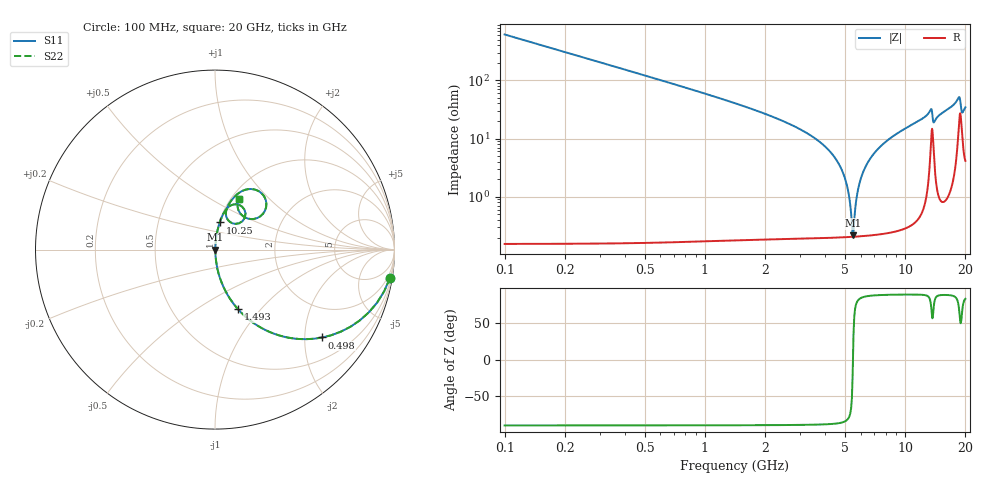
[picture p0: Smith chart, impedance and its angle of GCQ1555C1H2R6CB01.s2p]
!Murata Part Number: GCQ1555C1H2R6CB01
!These Parameters are Measured in Series Mode Connection
!Data Generated on Jan 08, 2026
!  o--ll--o
!Port1  Port2
!  o------o
!Operation Temp=25[degC], DC Bias Voltage=0[V]
!Freq. Start=100[MHz] Stop=20[GHz] 401[Steps]
# Hz S RI R 50
!Freq.(Hz) S11(Real) S11(Imag) S21(Real) S21(Imag) S12(Real) S12(Imag) S22(Real) S22(Imag)
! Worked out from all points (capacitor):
!   401 points, 100 MHz to 20 GHz, reference 50 ohm
!   read as one part in series: C = 2.6 pF near 199.5 MHz
!   lowest |Z| = 217 mohm at 5.473 GHz (marker M1)
!   series resonance near 5.49 GHz, so ESL is about 320 pH
!   S11 on the Smith chart (normalised r, x): 100 MHz: 1, -12; 498 MHz: 1.00, -2.44; 1.493 GHz: 1.00, -0.76; 10.25 GHz: 1.01, +0.31; 20 GHz: 1.08, +0.68
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1e8  0.974 -0.1592  0.026 0.1592  0.026 0.1592  0.974 -0.1592
2.99e8  0.8063 -0.3948  0.1937 0.3948  0.1937 0.3948  0.8063 -0.3948
4.98e8  0.5976 -0.4897  0.4024 0.4897  0.4024 0.4897  0.5976 -0.4897
9.4575e8  0.2834 -0.4493  0.7166 0.4493  0.7166 0.4493  0.2834 -0.4493
1.493e9  0.1272 -0.3309  0.8728 0.3309  0.8728 0.3309  0.1272 -0.3309
3.43325e9  0.0136 -0.1072  0.9864 0.1072  0.9864 0.1072  0.0136 -0.1072
4.876e9  0.00272 -0.0266  0.9973 0.0266  0.9973 0.0266  0.00272 -0.0266
5.1745e9  0.00221 -0.0132  0.9978 0.0132  0.9978 0.0132  0.00221 -0.0132
5.473e9  0.00206 -0.000683  0.9979 0.000683  0.9979 0.000683  0.00206 -0.000683
5.5725e9  0.00207 0.00336  0.9979 -0.00336  0.9979 -0.00336  0.00207 0.00336
5.7715e9  0.0022 0.0112  0.9978 -0.0112  0.9978 -0.0112  0.0022 0.0112
5.9705e9  0.00245 0.0189  0.9975 -0.0189  0.9975 -0.0189  0.00245 0.0189
6.7665e9  0.00443 0.0474  0.9956 -0.0474  0.9956 -0.0474  0.00443 0.0474
8.06e9  0.0103 0.0887  0.9897 -0.0887  0.9897 -0.0887  0.0103 0.0887
1.005e10  0.0246 0.1457  0.9754 -0.1457  0.9754 -0.1457  0.0246 0.1457
1.0249e10  0.0264 0.1512  0.9736 -0.1512  0.9736 -0.1512  0.0264 0.1512
1.338325e10  0.1261 0.2511  0.8739 -0.2511  0.8739 -0.2511  0.1261 0.2511
1.388075e10  0.0845 0.1534  0.9155 -0.1534  0.9155 -0.1534  0.0845 0.1534
1.67165e10  0.1098 0.2955  0.8902 -0.2955  0.8902 -0.2955  0.1098 0.2955
1.87065e10  0.2862 0.2569  0.7138 -0.2569  0.7138 -0.2569  0.2862 0.2569
1.9204e10  0.1583 0.1848  0.8417 -0.1848  0.8417 -0.1848  0.1583 0.1848
2e10  0.133 0.2842  0.867 -0.2842  0.867 -0.2842  0.133 0.2842
